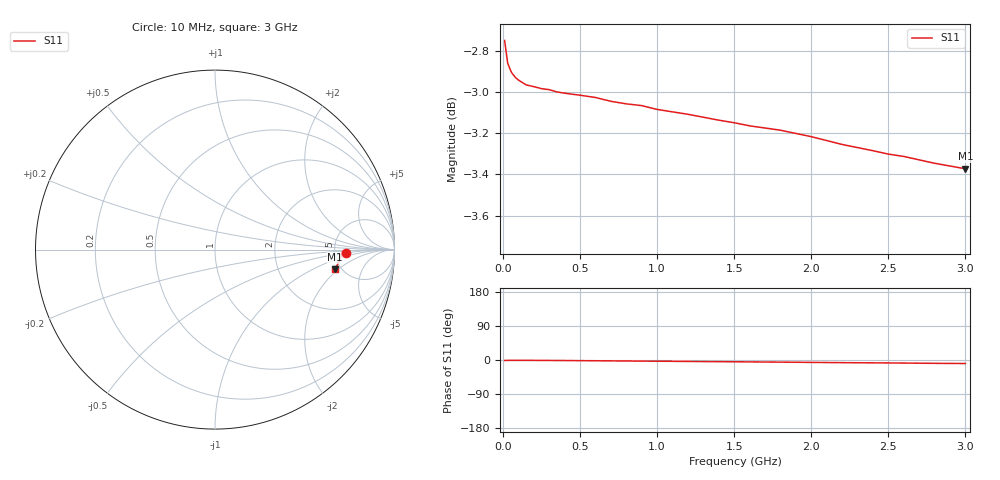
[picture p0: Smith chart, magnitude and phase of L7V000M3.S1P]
! SIEMENS Small Signal Semiconductors
! BAR14-1
! Si PIN Diode in SOT23
! IF = 0.3 mA
! S-Parameters:  July  1992
# GHz  S  MA  R  50
!  f  S11
! GHz  MAG  ANG
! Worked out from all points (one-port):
!   31 points, 10 MHz to 3 GHz, reference 50 ohm
!   lowest |S11| = -3.4 dB at 3 GHz (marker M1), VSWR 5.22, Z = 222 - j90.3 ohm
!   |S11| at or under -10 dB: nowhere
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0.01  0.7287 -1.3
0.03  0.7195 -1.0
0.05  0.7164 -0.9
0.06  0.7153 -0.9
0.08  0.7138 -0.9
0.1  0.7127 -0.9
0.15  0.7108 -0.9
0.25  0.7093 -1.1
0.3  0.7089 -1.2
0.35  0.708 -1.3
0.4  0.7075 -1.4
0.45  0.7071 -1.6
0.5  0.7067 -1.7
0.6  0.7058 -2.0
0.7  0.7043 -2.3
0.8  0.7033 -2.6
0.9  0.7026 -2.9
1  0.7011 -3.2
1.2  0.6992 -3.8
1.6  0.6947 -5.0
1.8  0.693 -5.6
2  0.6905 -6.3
2.2  0.6875 -7.0
2.4  0.6851 -7.5
2.5  0.6838 -7.8
2.6  0.6829 -8.1
2.8  0.6803 -8.8
3  0.6782 -9.3
